{attribute 'pack_mode' := '1'}
TYPE ST_OutputArgInfoAndData :
STRUCT
	nNumberOfOutputArguments: UDINT; // determined amount of output parameters
	nReserved: ARRAY[1..4] OF BYTE; // Reserved padding
	stOutputArgInfo: ARRAY[1..1] OF ST_UAMethodArgInfo; // number of output parameters - M_Mul has 1 output parameter 
	pro: DINT;
END_STRUCT
END_TYPE
